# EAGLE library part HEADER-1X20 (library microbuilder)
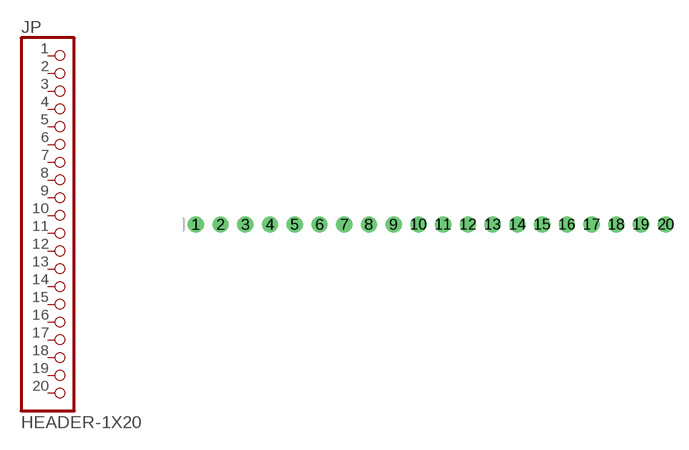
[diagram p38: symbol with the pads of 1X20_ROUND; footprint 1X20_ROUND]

Designator prefix JP

## HEADER-1X20ROUND  [1X20_ROUND]
1  1  pas
2  2  pas
3  3  pas
4  4  pas
5  5  pas
6  6  pas
7  7  pas
8  8  pas
9  9  pas
10  10  pas
11  11  pas
12  12  pas
13  13  pas
14  14  pas
15  15  pas
16  16  pas
17  17  pas
18  18  pas
19  19  pas
20  20  pas

## Footprint 1X20_ROUND (pad centres in mm)
drill 1 pad 1.676: 1 -24.13,0; 2 -21.59,0; 3 -19.05,0; 4 -16.51,0; 5 -13.97,0; 6 -11.43,0; 7 -8.89,0; 8 -6.35,0; 9 -3.81,0; 10 -1.27,0; 11 1.27,0; 12 3.81,0; 13 6.35,0; 14 8.89,0; 15 11.43,0; 16 13.97,0; 17 16.51,0; 18 19.05,0; 19 21.59,0; 20 24.13,0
